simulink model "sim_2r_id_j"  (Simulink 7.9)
settings: Solver=ode45  StartTime=0.0  StopTime=10  RelTol=1e-3
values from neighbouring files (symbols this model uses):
  m = 1    [mechanical_system.m]
  s = Lv/norm(Lv)    [pkm1.m]
undefined symbols (not defined in the file or in its folder): deg, kg, mN, N, rad
libraries: mblibv1 x12

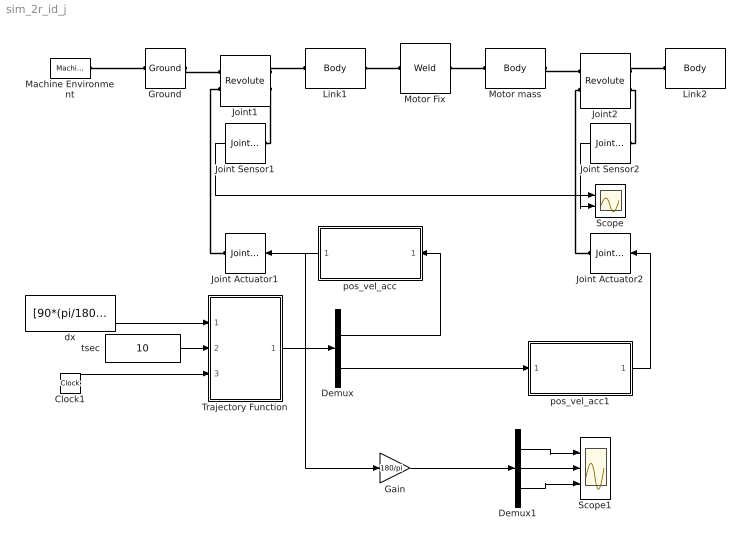
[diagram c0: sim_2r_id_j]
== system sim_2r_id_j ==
  Clock1 : Clock
  Demux : Demux  Outputs=2
  Demux1 : Demux  Outputs=3
  Gain : Gain  Gain=180/pi
  Ground : mblibv1/Bodies/Ground  UpdateFromCAD=off  LeftPortType=env  RightPortType=workingframe  PhysicalDomain=Mechanical  DialogClass=GroundBlock  CoordPosition=[0 0 0]  CoordPositionUnits=m  StateVectorMgrId=2  MachineId=[3 0]  ShowEnvPort=on
  Joint Actuator1 : mblibv1/Sensors &  Actuators/Joint Actuator  UpdateFromCAD=off  PhysicalDomain=Mechanical  PortType=blob  ActuationStyle=Motion  AngleUnits=rad  ArcVelocityUnits=rad/s  ArcAccelerationUnits=rad/s^2  CoordPositionUnits=m  VelocityUnits=m/s  AccelerationUnits=m/s^2  ForceUnits=N  TorqueUnits=N*m  ActiveIO=on  Width=3  DialogClass=MechanicalActuatorBlock  Primitive=R1  ReferenceFrame=Absolute (World)
  Joint Actuator2 : mblibv1/Sensors &  Actuators/Joint Actuator  UpdateFromCAD=off  PhysicalDomain=Mechanical  PortType=blob  ActuationStyle=Motion  AngleUnits=rad  ArcVelocityUnits=rad/s  ArcAccelerationUnits=rad/s^2  CoordPositionUnits=m  VelocityUnits=m/s  AccelerationUnits=m/s^2  ForceUnits=N  TorqueUnits=N*m  ActiveIO=on  Width=3  DialogClass=MechanicalActuatorBlock  Primitive=R1  ReferenceFrame=Absolute (World)
  Joint Sensor1 : mblibv1/Sensors &  Actuators/Joint Sensor  UpdateFromCAD=off  PhysicalDomain=Mechanical  PortType=blob  Muxed=on  Pose=off  Angle=off  AngleUnits=deg  ArcVelocity=off  ArcVelocityUnits=deg/s  ArcAcceleration=off  ArcAccelerationUnits=deg/s^2  CoordPosition=on  CoordPositionUnits=m  Velocity=off  VelocityUnits=m/s  Acceleration=off  AccelerationUnits=m/s^2  Quaternion=on  QuaternionDT=off  QuaternionDDT=off  QuaternionUnits=off  OutputVector=[1]  ActiveIO=on  Width=1  DialogClass=MechanicalSensorBlock  Primitive=R1  Force=off  ForceUnits=N  Torque=on  TorqueUnits=mN*m  ReferenceFrame=Absolute (World)  ReactionSensedSide=Base  ReactionReferenceFrame=Absolute (World)  ReactionForce=off  ReactionForceUnits=N  ReactionMoment=off  ReactionMomentUnits=N*m
  Joint Sensor2 : mblibv1/Sensors &  Actuators/Joint Sensor  UpdateFromCAD=off  PhysicalDomain=Mechanical  PortType=blob  Muxed=on  Pose=off  Angle=off  AngleUnits=deg  ArcVelocity=off  ArcVelocityUnits=deg/s  ArcAcceleration=off  ArcAccelerationUnits=deg/s^2  CoordPosition=on  CoordPositionUnits=m  Velocity=off  VelocityUnits=m/s  Acceleration=off  AccelerationUnits=m/s^2  Quaternion=on  QuaternionDT=off  QuaternionDDT=off  QuaternionUnits=off  OutputVector=[1]  ActiveIO=on  Width=1  DialogClass=MechanicalSensorBlock  Primitive=R1  Force=off  ForceUnits=N  Torque=on  TorqueUnits=mN*m  ReferenceFrame=Absolute (World)  ReactionSensedSide=Base  ReactionReferenceFrame=Absolute (World)  ReactionForce=off  ReactionForceUnits=N  ReactionMoment=off  ReactionMomentUnits=N*m
  Joint1 : mblibv1/Joints/Revolute  LConnTagsString=__newl0|SA1  RConnTagsString=__newr0|SA1  UpdateFromCAD=off  NumSAPorts=2  CutJoint=off  MarkAsCut=off  Primitives=prismatic  PrimitiveProps=R1$World$[0 0 1]$revolute  DialogClass=JointBlock  R1Axis=[0 0 1]
  Joint2 : mblibv1/Joints/Revolute  LConnTagsString=__newl0|SA1  RConnTagsString=__newr0|SA1  UpdateFromCAD=off  NumSAPorts=2  CutJoint=off  MarkAsCut=off  Primitives=prismatic  PrimitiveProps=R1$World$[0 0 1]$revolute  DialogClass=JointBlock  R1Axis=[0 0 1]
  Link1 : mblibv1/Bodies/Body  LConnTagsString=CS1  RConnTagsString=CS2  UpdateFromCAD=off  DialogClass=MechanicalBodyBlock  Mass=0.071  MassUnits=kg  InertiaUnits=kg*m^2  Inertia=[0 0 0; 0 0 0; 0 0 0.000089395]  Shape=Cylinder  ShapeDims=[1 1]  ShapeUnits=m  ShapeUse=false  Density=1  DensityUnits=kg/m^3  DensityUse=false  GraphicsMode=MACHINE_DEFAULT  BodyColorSelMode=MACHINE_DEFAULT  BodyColor=[1 0 0]  AttachedToCS=CG  CG=Left$CG$[0.0373 0 0]$CS1$CS1$m$[0 0 0]$Euler X-Y-Z$deg$WORLD$false$none  WorkingFrames=Left$CS1$[0 0 0]$World$World$m$[0 0 0]$Euler X-Y-Z$deg$WORLD$true$none#Right$CS2$[0.1 0 0]$World$World$m$[0 0 0]$Euler X-Y-Z$deg$WORLD$true$none  CGPos=[0.0373 0 0]  CGRot=[0 0 0]  CS0Pos=[]  CS0Rot=[]  CS1Pos=[0 0 0]  CS1Rot=[0 0 0]  CS2Pos=[0.1 0 0]  CS2Rot=[0 0 0]  CS3Pos=[]  CS3Rot=[]  CS4Pos=[]  CS4Rot=[]  CS5Pos=[]  CS5Rot=[]  CS6Pos=[]  CS6Rot=[]  CS7Pos=[]  CS7Rot=[]  CS8Pos=[]  CS8Rot=[]  CS9Pos=[]  CS9Rot=[]  CS10Pos=[]  CS10Rot=[]  CS11Pos=[]  CS11Rot=[]  CS12Pos=[]  CS12Rot=[]  CS13Pos=[]  CS13Rot=[]  CS14Pos=[]  CS14Rot=[]  CS15Pos=[]  CS15Rot=[]  CS16Pos=[]  CS16Rot=[]  CS17Pos=[]  CS17Rot=[]  CS18Pos=[]  CS18Rot=[]  CS19Pos=[]  CS19Rot=[]  CS20Pos=[]  CS20Rot=[]
  Link2 : mblibv1/Bodies/Body  LConnTagsString=CS1  UpdateFromCAD=off  DialogClass=MechanicalBodyBlock  Mass=0.1  MassUnits=kg  InertiaUnits=kg*m^2  Inertia=[0 0 0; 0 0 0; 0 0 0.000109864]  Shape=Cylinder  ShapeDims=[1 1]  ShapeUnits=m  ShapeUse=false  Density=1  DensityUnits=kg/m^3  DensityUse=false  GraphicsMode=MACHINE_DEFAULT  BodyColorSelMode=MACHINE_DEFAULT  BodyColor=[1 0 0]  AttachedToCS=CG  CG=Left$CG$[0.04168 0 0]$CS1$CS1$m$[0 0 0]$Euler X-Y-Z$deg$WORLD$false$none  WorkingFrames=Left$CS1$[0.1 0 0]$World$World$m$[0 0 0]$Euler X-Y-Z$deg$WORLD$true$none#Right$CS2$[0.2 0 0]$World$World$m$[0 0 0]$Euler X-Y-Z$deg$WORLD$false$none  CGPos=[0.04168 0 0]  CGRot=[0 0 0]  CS0Pos=[]  CS0Rot=[]  CS1Pos=[0.1 0 0]  CS1Rot=[0 0 0]  CS2Pos=[0.2 0 0]  CS2Rot=[0 0 0]  CS3Pos=[]  CS3Rot=[]  CS4Pos=[]  CS4Rot=[]  CS5Pos=[]  CS5Rot=[]  CS6Pos=[]  CS6Rot=[]  CS7Pos=[]  CS7Rot=[]  CS8Pos=[]  CS8Rot=[]  CS9Pos=[]  CS9Rot=[]  CS10Pos=[]  CS10Rot=[]  CS11Pos=[]  CS11Rot=[]  CS12Pos=[]  CS12Rot=[]  CS13Pos=[]  CS13Rot=[]  CS14Pos=[]  CS14Rot=[]  CS15Pos=[]  CS15Rot=[]  CS16Pos=[]  CS16Rot=[]  CS17Pos=[]  CS17Rot=[]  CS18Pos=[]  CS18Rot=[]  CS19Pos=[]  CS19Rot=[]  CS20Pos=[]  CS20Rot=[]
  Machine Environment : mblibv1/Bodies/Machine Environment  PortType=env  PhysicalDomain=Mechanical  DialogTemplateClass=MECH.MachineEnvironment  SyncWhenCopied=off  Gravity=[0 -9.81 0]  GravityUnits=m/s^2  GravityAsSignal=off  Dimensionality=Auto-detect  AnalysisType=Forward dynamics  LinearAssemblyTolerance=1e-3  LinearAssemblyToleranceUnits=m  AngularAssemblyTolerance=1e-3  AngularAssemblyToleranceUnits=rad  ConstraintSolverType=Stabilizing  ConstraintRelTolerance=1e-4  ConstraintAbsTolerance=1e-4  UseRobustSingularityHandling=off  RedundancyAnalysisToleranceType=Automatically select tolerance  RedundancyAnalysisTolerance=1e-14  StatePerturbationType=Fixed  PerturbationSize=1e-5  VisualizeMachine=on  BodyVisualizationType=Use model default body geometries  BodyColorSelMode=Use model default  DefaultBodyColor=[1 0 0]
  Motor Fix : mblibv1/Joints/Weld  LConnTagsString=__newl0  RConnTagsString=__newr0  UpdateFromCAD=off  NumSAPorts=0  CutJoint=off  MarkAsCut=off  Primitives=weld  PrimitiveProps=W$WORLD$[0 0 0]$weld  DialogClass=JointBlock  WAxis=[0 0 0]
  Motor mass : mblibv1/Bodies/Body  LConnTagsString=CS1  RConnTagsString=CS2  UpdateFromCAD=off  DialogClass=MechanicalBodyBlock  Mass=0.292  MassUnits=kg  InertiaUnits=kg*m^2  Inertia=[0 0 0; 0 0 0; 0 0 0]  Shape=Cylinder  ShapeDims=[1 1]  ShapeUnits=m  ShapeUse=false  Density=1  DensityUnits=kg/m^3  DensityUse=false  GraphicsMode=MACHINE_DEFAULT  BodyColorSelMode=MACHINE_DEFAULT  BodyColor=[1 0 0]  AttachedToCS=CG  CG=Left$CG$[0.1 0 0]$WORLD$WORLD$m$[0 0 0]$Euler X-Y-Z$deg$WORLD$false$none  WorkingFrames=Left$CS1$[0.1 0 0]$World$World$m$[0 0 0]$Euler X-Y-Z$deg$WORLD$true$none#Right$CS2$[0.1 0 0]$World$World$m$[0 0 0]$Euler X-Y-Z$deg$WORLD$true$none  CGPos=[0.1 0 0]  CGRot=[0 0 0]  CS0Pos=[]  CS0Rot=[]  CS1Pos=[0.1 0 0]  CS1Rot=[0 0 0]  CS2Pos=[0.1 0 0]  CS2Rot=[0 0 0]  CS3Pos=[]  CS3Rot=[]  CS4Pos=[]  CS4Rot=[]  CS5Pos=[]  CS5Rot=[]  CS6Pos=[]  CS6Rot=[]  CS7Pos=[]  CS7Rot=[]  CS8Pos=[]  CS8Rot=[]  CS9Pos=[]  CS9Rot=[]  CS10Pos=[]  CS10Rot=[]  CS11Pos=[]  CS11Rot=[]  CS12Pos=[]  CS12Rot=[]  CS13Pos=[]  CS13Rot=[]  CS14Pos=[]  CS14Rot=[]  CS15Pos=[]  CS15Rot=[]  CS16Pos=[]  CS16Rot=[]  CS17Pos=[]  CS17Rot=[]  CS18Pos=[]  CS18Rot=[]  CS19Pos=[]  CS19Rot=[]  CS20Pos=[]  CS20Rot=[]
  Scope : Scope  NumInputPorts=2
  Scope1 : Scope  NumInputPorts=3
  Trajectory Function : MATLAB Function  TreatAsAtomicUnit=on
  dx : Constant  Value=[90*(pi/180), 0]'
  pos_vel_acc : Subsystem
  pos_vel_acc1 : Subsystem
  tsec : Constant  Value=10
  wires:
  Joint Sensor1/1 -> Scope/1
  Joint Sensor2/1 -> Scope/2
  Clock1/1 -> Trajectory Function/3(tout)
  tsec/1 -> Trajectory Function/2(tsec)
  dx/1 -> Trajectory Function/1(dx)
  pos_vel_acc1/1(Motion2) -> Joint Actuator2/1
  Demux/1 -> pos_vel_acc/1(In1)
  Demux/2 -> pos_vel_acc1/1(In1)
  Trajectory Function/1(xd) -> Demux/1
  pos_vel_acc/1(Motion1) -> Joint Actuator1/1, Gain/1
  Demux1/1 -> Scope1/1
  Demux1/2 -> Scope1/2
  Demux1/3 -> Scope1/3
  Gain/1 -> Demux1/1
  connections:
  Machine Environment/RConn1 -- Ground/LConn1
  Joint1/RConn1 -- Link1/LConn1
  Ground/RConn1 -- Joint1/LConn1
  Link1/RConn1 -- Motor Fix/LConn1
  Motor Fix/RConn1 -- Motor mass/LConn1
  Motor mass/RConn1 -- Joint2/LConn1
  Joint2/RConn1 -- Link2/LConn1
  Joint1/RConn2 -- Joint Sensor1/LConn1
  Joint2/RConn2 -- Joint Sensor2/LConn1
  Joint1/LConn2 -- Joint Actuator1/RConn1
  Joint2/LConn2 -- Joint Actuator2/RConn1

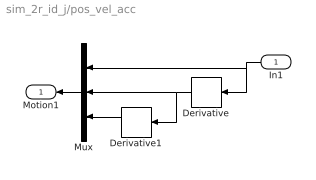
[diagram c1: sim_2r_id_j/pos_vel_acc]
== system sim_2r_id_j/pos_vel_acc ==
  In1 : Inport
  Derivative : Derivative
  Derivative1 : Derivative
  Mux : Mux  Inputs=3
  Motion1 : Outport
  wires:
  Derivative/1 -> Mux/2, Derivative1/1
  Derivative1/1 -> Mux/3
  In1/1 -> Mux/1, Derivative/1
  Mux/1 -> Motion1/1

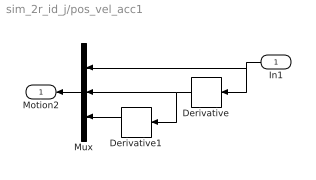
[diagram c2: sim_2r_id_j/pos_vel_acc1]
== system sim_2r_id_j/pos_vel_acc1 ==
  In1 : Inport
  Derivative : Derivative
  Derivative1 : Derivative
  Mux : Mux  Inputs=3
  Motion2 : Outport
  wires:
  Derivative/1 -> Mux/2, Derivative1/1
  Derivative1/1 -> Mux/3
  In1/1 -> Mux/1, Derivative/1
  Mux/1 -> Motion2/1

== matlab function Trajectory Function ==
function xd = fcn(dx, tsec, tout)

MAX_CH=2;       % Two Actuators %
D2R=pi/180;

% Initializing Variables %
xd=zeros(MAX_CH,1);
x0=D2R*[0,0]';



    [c] = coeff_3rd(x0, zeros(MAX_CH,1), x0+dx, zeros(MAX_CH,1), tsec);
    for ch=1:MAX_CH
        xd(ch,1)=c(ch,1)+c(ch,2)*tout+c(ch,3)*tout^2+c(ch,4)*tout^3;    
    end

function [c] = coeff_3rd(sp, sv, ep, ev, tsec)
MAX_CH=2;
c=zeros(MAX_CH,4);
for ch=1:MAX_CH
    c(ch,1)=sp(ch,1);
    c(ch,2)=sv(ch,1);
    c(ch,3)=(3.0*(ep(ch,1)-sp(ch,1))-(2.0*sv(ch,1)+ev(ch,1))*tsec)/(tsec*tsec);
    c(ch,4)=(-2.0*(ep(ch,1)-sp(ch,1))+(sv(ch,1)+ev(ch,1))*tsec)/(tsec*tsec*tsec);
end
